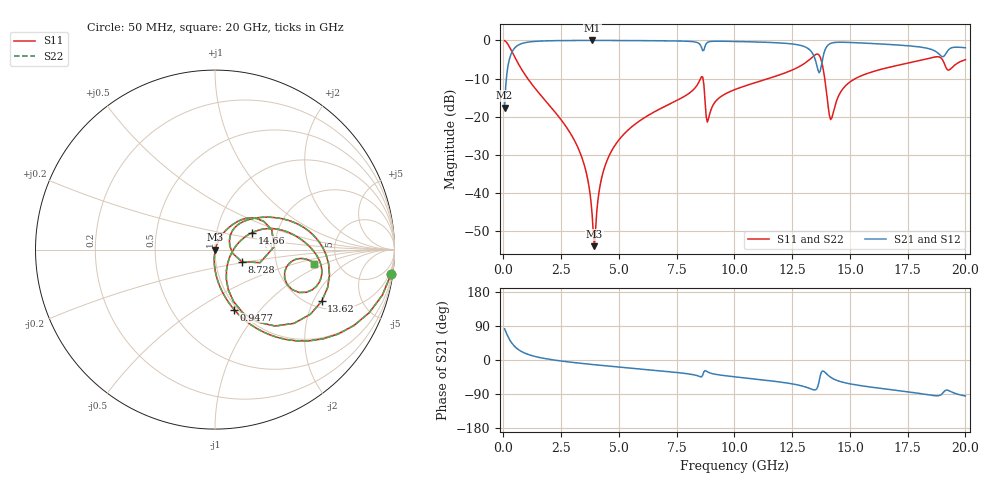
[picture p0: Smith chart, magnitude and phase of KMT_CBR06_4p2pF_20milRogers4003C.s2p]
! Data measured by Modelithics Inc. support@modelithics.com 813-866-6335
! KEMET CBR0603 4.2pF, Pad Width= 0.851mm, Pad Length= 0.64mm, Pad Gap= 0.62mm, 20mil Rogers 4003C substrate Data, January 2022
# hz S ma R 50
! 2 Port Network Data from SP1.SP block
! freq  magS11  angS11  magS21  angS21  magS12  angS12  magS22  angS22
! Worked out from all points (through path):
!   401 points, 50 MHz to 20 GHz, reference 50 ohm
!   highest |S21| = -0.02 dB at 3.841 GHz (marker M1); lowest = -17.6 dB at 50 MHz (marker M2)
!   group delay of S21, straight-line fit = 15.7 ps
!   lowest |S11| = -53.9 dB at 3.94 GHz (marker M3), VSWR 1.00, Z = 50.2 - j0.0131 ohm
!   |S11| at or under -10 dB: 1.05 GHz to 8.533 GHz (7.484 GHz wide, 156 % of centre); 8.637 GHz to 11.47 GHz (2.832 GHz wide, 28.2 % of centre); 13.91 GHz to 15.24 GHz (1.331 GHz wide, 9.13 % of centre)
!   |S22| runs from -53.9 to -0.1 dB; largest |S21 - S12| = 0
!   S11 on the Smith chart (normalised r, x): 50 MHz: 1, -15; 947.8 MHz: 0.96, -0.73; 8.728 GHz: 1.33, -0.18; 13.62 GHz: 2.27, -2.33; 14.66 GHz: 1.48, +0.29; 20 GHz: 3.34, -0.75
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5e7  0.9912 -7.7  0.1319 82.3  0.1319 82.3  0.9912 -7.7
3.4925e8  0.7297 -44.2  0.683 45.8  0.683 45.8  0.7297 -44.2
9.4775e8  0.3504 -72.3  0.9355 17.5  0.9355 17.5  0.3504 -72.3
3.391625e9  0.02942 -95.4  0.9976 -9.0  0.9976 -9.0  0.02942 -95.4
3.690875e9  0.01282 -92.3  0.9979 -10.9  0.9979 -10.9  0.01282 -92.3
3.8405e9  0.005187 -79.6  0.9979 -11.8  0.9979 -11.8  0.005187 -79.6
3.94025e9  0.00201 -3.7  0.9979 -12.5  0.9979 -12.5  0.00201 -3.7
4.2395e9  0.01518 68.0  0.9977 -14.2  0.9977 -14.2  0.01518 68.0
4.688375e9  0.03594 69.7  0.997 -16.8  0.997 -16.8  0.03594 69.7
6.73325e9  0.1247 60.3  0.989 -28.3  0.989 -28.3  0.1247 60.3
8.52875e9  0.3143 29.8  0.8669 -44.3  0.8669 -44.3  0.3143 29.8
8.72825e9  0.1624 -24.3  0.8376 -27.9  0.8376 -27.9  0.1624 -24.3
8.877875e9  0.09416 31.5  0.9551 -32.7  0.9551 -32.7  0.09416 31.5
1.0025e10  0.227 44.2  0.9681 -44.4  0.9681 -44.4  0.227 44.2
1.336662e10  0.6016 0.9  0.6869 -77.6  0.6869 -77.6  0.6016 0.9
1.3616e10  0.6604 -25.9  0.4099 -69.1  0.4099 -69.1  0.6604 -25.9
1.38155e10  0.4664 -59.8  0.57 -29.0  0.57 -29.0  0.4664 -59.8
1.416462e10  0.09173 -26.7  0.9123 -45.5  0.9123 -45.5  0.09173 -26.7
1.466338e10  0.2251 24.5  0.946 -58.2  0.946 -58.2  0.2251 24.5
1.670825e10  0.4445 10.8  0.8845 -77.8  0.8845 -77.8  0.4445 10.8
1.90025e10  0.5614 -25.1  0.6116 -88.3  0.6116 -88.3  0.5614 -25.1
2e10  0.5585 -8.0  0.8004 -95.0  0.8004 -95.0  0.5585 -8.0
